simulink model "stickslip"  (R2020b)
settings: Solver=ode5  StartTime=0.0  StopTime=5  FixedStep=0.001  RelTol=1e-3  AbsTol=1e-3  EnableMultiTasking=on
model workspace (MAT data in the model file):
  FGR = 7
  Tv = 0.1
  c = 60
  dF = 3
  m = 1
  vB = 0.1
undefined symbols (not defined in the file or in its folder): sgn

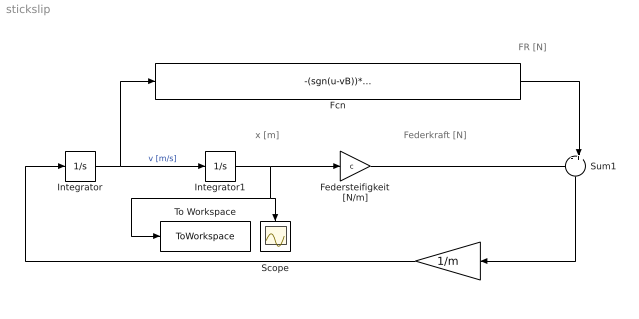
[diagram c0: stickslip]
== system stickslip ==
  note: x [m]
  note: Federkraft [N]
  note: FR [N]
  "  " : Gain  Gain=1/m  SaturateOnIntegerOverflow=on
  Fcn : Fcn  Expr=-(sgn(u-vB))*(FGR+dF*exp(-abs(u-vB)/Tv))
  Federsteifigkeit [N/m] : Gain  Gain=c  SaturateOnIntegerOverflow=on
  Integrator : Integrator
  Integrator1 : Integrator
  Scope : Scope
  Sum1 : Sum  Inputs=-+|  SaturateOnIntegerOverflow=on
  To Workspace : ToWorkspace  VariableName=out  SaveFormat=Timeseries  SampleTime=-1
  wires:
  Federsteifigkeit [N/m]/1 -> Sum1/1
  Integrator/1 -> Integrator1/1, Fcn/1  "v [m/s]"
  Fcn/1 -> Sum1/2
  Integrator1/1 -> To Workspace/1, Scope/1, Federsteifigkeit [N/m]/1
  "  "/1 -> Integrator/1
  Sum1/1 -> "  "/1
